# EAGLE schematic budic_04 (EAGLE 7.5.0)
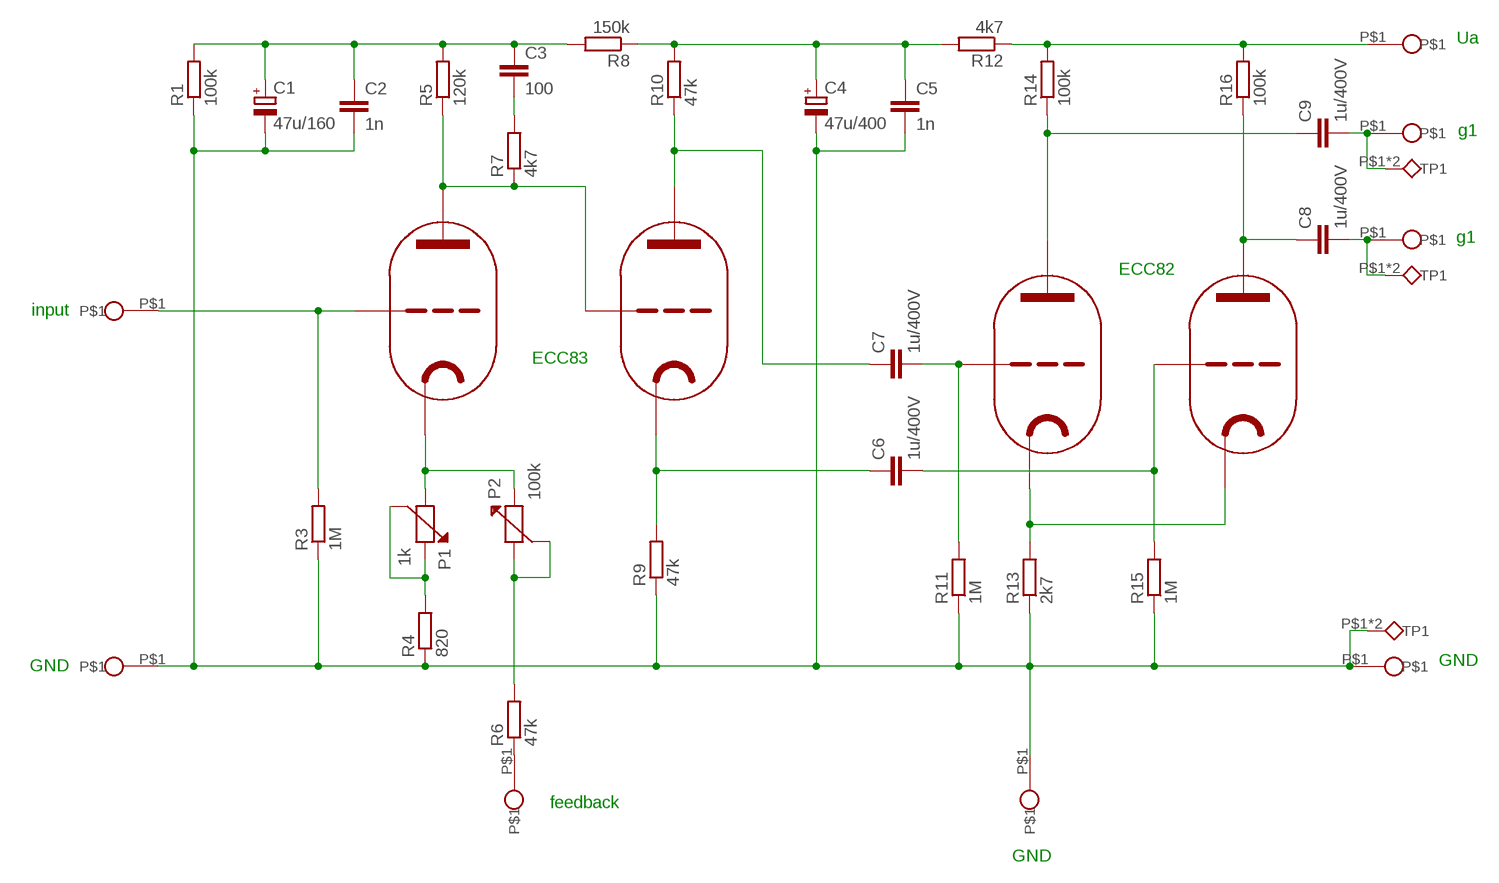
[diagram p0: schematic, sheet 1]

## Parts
C1  47u/160  CPOL-EUE5-10.5  [E5-10,5]
C2  1n  C-EU050-024X044  [C050-024X044]
C3  100  C-EU050-024X044  [C050-024X044]
C4  47u/400  CPOL-EUE7.5-18  [E7,5-18]
C5  1n  C-EU050-024X044  [C050-024X044]
C6  1u/400V  C-EU150-091X182  [C150-091X182]
C7  1u/400V  C-EU150-091X182  [C150-091X182]
C8  1u/400V  C-EU150-091X182  [C150-091X182]
C9  1u/400V  C-EU150-091X182  [C150-091X182]
E1  ECC83  ECC82_218MM  [NOVAL03]
E2  ECC82  ECC82_218MM  [NOVAL03]
P1  1k  P10V  [PT10V]
P2  100k  P10V  [PT10V]
R1  100k  R-EU_0207/10  [0207/10]
R3  1M  R-EU_0207/10  [0207/10]
R4  820  R-EU_0207/10  [0207/10]
R5  120k  R-EU_0207/10  [0207/10]
R6  47k  R-EU_0207/10  [0207/10]
R7  4k7  R-EU_0207/10  [0207/10]
R8  150k  R-EU_0207/10  [0207/10]
R9  47k  R-EU_0207/10  [0207/10]
R10  47k  R-EU_0207/10  [0207/10]
R11  1M  R-EU_0207/10  [0207/10]
R12  4k7  R-EU_0207/10  [0207/10]
R13  2k7  R-EU_0207/10  [0207/10]
R14  100k  R-EU_0207/10  [0207/10]
R15  1M  R-EU_0207/10  [0207/10]
R16  100k  R-EU_0207/10  [0207/10]
U$1  TESTPIN  [TESTPIN2]
U$2  TESTPIN  [TESTPIN2]
U$3  PIN  [PIN]
U$4  TESTPIN  [TESTPIN2]
U$14  PIN  [PIN]
U$38  input  PIN  [PIN]
U$40  PIN  [PIN]
U$42  PIN  [PIN]
U$58  PIN  [PIN]
U$62  PIN  [PIN]
UA  Ua  PIN  [PIN]

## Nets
A1: C8.1 E2.P$1(A) R16.1
GND: C1.- C2.2 C4.- C5.2 R1.1 R3.1 R4.1 R9.1 R11.1 R13.1 R15.1 U$4.P$1(TP1) U$4.P$2(TP1) U$40.P$1 U$58.P$1 U$62.P$1
N$1: C9.2 U$1.P$1(TP1) U$1.P$2(TP1) U$3.P$1
N$2: E1.P$2(G1) E1.P$6(A) R5.1 R7.1
N$3: C8.2 U$2.P$1(TP1) U$2.P$2(TP1) U$14.P$1
N$4: C4.+ C5.1 R8.1 R10.2 R12.2
N$5: P1.2 P1.3 R4.2
N$9: E1.P$7(G1) R3.2 U$38.P$1
N$10: E1.P$8(K) P1.1 P2.2
N$11: C3.2 R7.2
N$14: C7.1 E1.P$1(A) R10.1
N$15: C1.+ C2.1 C3.1 R1.2 R5.2 R8.2
N$18: E2.P$3(K) E2.P$8(K) R13.2
N$19: R12.1 R14.2 R16.2 UA.P$1
N$20: C9.1 E2.P$6(A) R14.1
N$22: C7.2 E2.P$7(G1) R11.2
N$30: C6.1 E1.P$3(K) R9.2
N$31: C6.2 E2.P$2(G1) R15.2
N$39: P2.1 P2.3 R6.2
N$40: R6.1 U$42.P$1

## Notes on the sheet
- Ua
- g1
- g1
- ECC82
- input
- ECC83
- GND
- GND
- feedback
- GND

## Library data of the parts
C1 C4 = rcl:CPOL-EU: POLARIZED CAPACITOR, European symbol
C2 C3 C5-C9 = rcl:C-EU: CAPACITOR, European symbol
E1 E2 = lampy03:ECC82_2
P1 P2 = lampy02:P10V
R1 R3-R16 = rcl:R-EU_: RESISTOR, European symbol
U$1 U$2 U$4 = lampy04:TESTPIN
U$3 U$14 U$38 U$40 U$42 U$58 U$62 UA = lampy02:PIN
